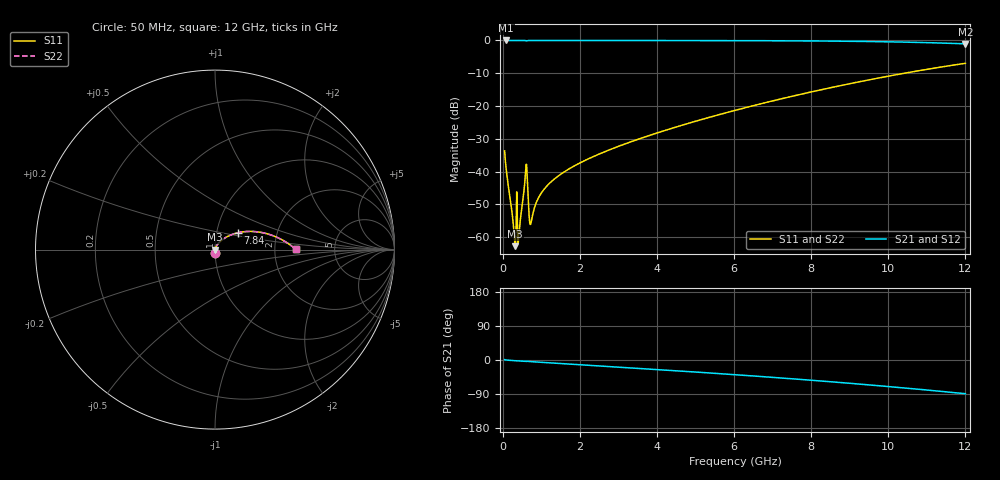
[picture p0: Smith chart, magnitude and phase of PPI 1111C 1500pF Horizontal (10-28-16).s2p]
# MHz S MA R 50
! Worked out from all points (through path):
!   1601 points, 50 MHz to 12 GHz, reference 50 ohm
!   highest |S21| = 0.00 dB at 87.34 MHz (marker M1); lowest = -1.0 dB at 12 GHz (marker M2)
!   group delay of S21, straight-line fit = 20.2 ps
!   lowest |S11| = -62.7 dB at 326.3 MHz (marker M3), VSWR 1.00, Z = 50.1 - j0.00941 ohm
!   |S11| at or under -10 dB: start of sweep to 10.42 GHz
!   |S22| runs from -62.7 to -7.0 dB; largest |S21 - S12| = 0
!   S11 on the Smith chart (normalised r, x): 50 MHz: 1.00, -0.04; 7.84 GHz: 1.26, +0.24; 12 GHz: 2.63, +0.02
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50  0.02077 -88.2  0.9995 0.9  0.9995 0.9  0.02077 -88.2
87.34375  0.01143 -88.0  0.9996 0.1  0.9996 0.1  0.01143 -88.0
274.0625  0.001607 -69.2  0.9994 -1.5  0.9994 -1.5  0.001607 -69.2
326.3438  0.000732 -7.4  0.9993 -1.9  0.9993 -1.9  0.000732 -7.4
363.6875  0.004918 8.9  0.9952 -2.2  0.9952 -2.2  0.004918 8.9
415.9688  0.0009933 35.6  0.9992 -2.5  0.9992 -2.5  0.0009933 35.6
445.8438  0.001578 56.2  0.9992 -2.7  0.9992 -2.7  0.001578 56.2
557.875  0.005491 66.3  0.9981 -3.5  0.9981 -3.5  0.005491 66.3
587.75  0.00887 54.9  0.9953 -3.9  0.9953 -3.9  0.00887 54.9
625.0938  0.01131 -13.4  0.9888 -3.5  0.9888 -3.5  0.01131 -13.4
699.7812  0.001707 -7.0  0.9983 -4.1  0.9983 -4.1  0.001707 -7.0
744.5938  0.001769 38.6  0.9987 -4.4  0.9987 -4.4  0.001769 38.6
908.9062  0.00379 68.1  0.9989 -5.5  0.9989 -5.5  0.00379 68.1
1125.5  0.005862 72.3  0.9988 -6.9  0.9988 -6.9  0.005862 72.3
1498.938  0.009091 73.1  0.9986 -9.2  0.9986 -9.2  0.009091 73.1
2044.156  0.01397 71.6  0.9984 -12.6  0.9984 -12.6  0.01397 71.6
4038.312  0.03949 61.8  0.997 -25.4  0.997 -25.4  0.03949 61.8
6025  0.08592 49.5  0.9934 -38.8  0.9934 -38.8  0.08592 49.5
7839.906  0.1563 36.7  0.984 -52.1  0.984 -52.1  0.1563 36.7
8019.156  0.1651 35.3  0.9825 -53.5  0.9825 -53.5  0.1651 35.3
10013.31  0.2864 19.0  0.9532 -70.2  0.9532 -70.2  0.2864 19.0
12000  0.4486 0.4  0.8876 -88.9  0.8876 -88.9  0.4486 0.4
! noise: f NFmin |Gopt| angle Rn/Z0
50  0.00038  0.8686  0.3026  0.0006222
1372  0.003943  0.6876  7.928  0.002441
2701  0.006435  0.6385  15.46  0.0033
4031  0.008716  0.6149  22.78  0.004054
5360  0.01093  0.6047  29.8  0.00479
6682  0.01315  0.6037  36.46  0.005564
8012  0.01548  0.6099  42.78  0.006433
9341  0.01797  0.6219  48.75  0.007445
1.067e+04  0.0207  0.6387  54.37  0.008662
1.2e+04  0.02375  0.6595  59.68  0.01017
